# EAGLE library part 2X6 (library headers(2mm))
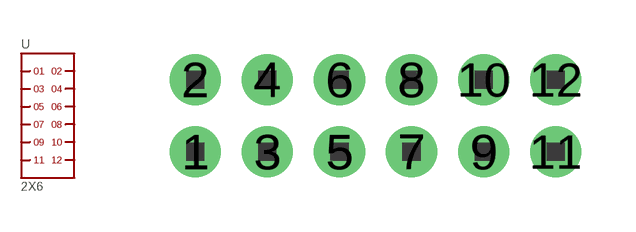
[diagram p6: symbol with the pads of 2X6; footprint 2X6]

Designator prefix -

## 2X6  [2X6]
1  1
2  2
3  3
4  4
5  5
6  6
7  7
8  8
9  9
10  10
11  11
12  12

## Footprint 2X6 (pad centres in mm)
drill 0.8 pad 1.422: 1 -5,-1; 2 -5,1; 3 -3,-1; 4 -3,1; 5 -1,-1; 6 -1,1; 7 1,-1; 8 1,1; 9 3,-1; 10 3,1; 11 5,-1; 12 5,1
